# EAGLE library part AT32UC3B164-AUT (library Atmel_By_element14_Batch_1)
MCU
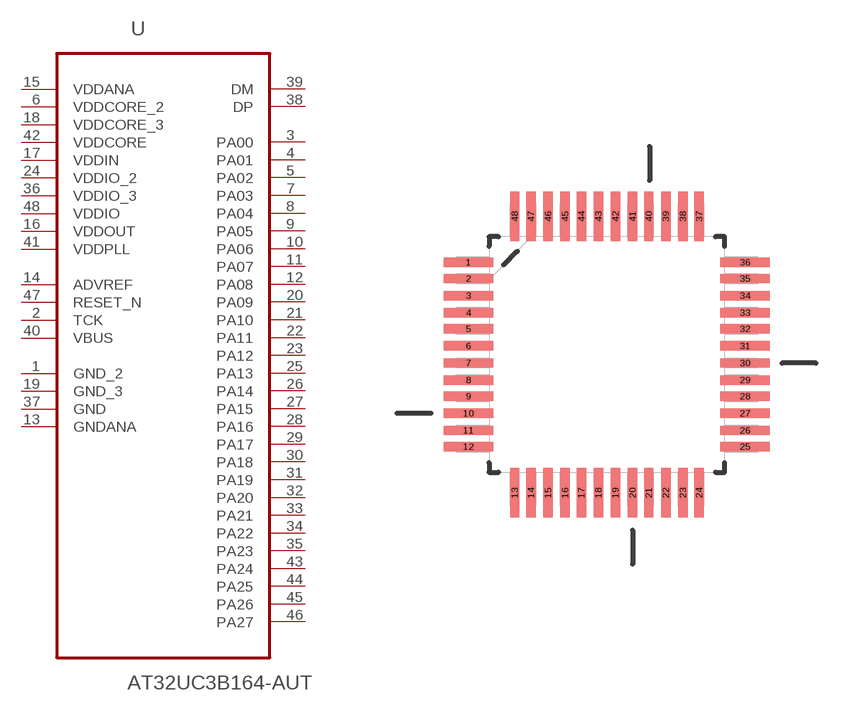
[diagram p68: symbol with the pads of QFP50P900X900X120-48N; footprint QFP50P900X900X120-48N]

Designator prefix U

## AT32UC3B164-AUT (DESCRIPTION: MCU; MPN: AT32UC3B164-AUT; OC_FARNELL: 1841642; OC_NEWARK: 12T1375; PACKAGE: QFP-48; SUPPLIER: Atmel)  [QFP50P900X900X120-48N]
1  GND_2  pas
2  TCK  in
3  PA00
4  PA01
5  PA02
6  VDDCORE_2  pwr
7  PA03
8  PA04
9  PA05
10  PA06
11  PA07
12  PA08
13  GNDANA  pas
14  ADVREF  in
15  VDDANA  pwr
16  VDDOUT  pwr
17  VDDIN  pwr
18  VDDCORE_3  pwr
19  GND_3  pas
20  PA09
21  PA10
22  PA11
23  PA12
24  VDDIO_2  pwr
25  PA13
26  PA14
27  PA15
28  PA16
29  PA17
30  PA18
31  PA19
32  PA20
33  PA21
34  PA22
35  PA23
36  VDDIO_3  pwr
37  GND  pas
38  DP
39  DM
40  VBUS  in
41  VDDPLL  pwr
42  VDDCORE  pwr
43  PA24
44  PA25
45  PA26
46  PA27
47  RESET_N  in
48  VDDIO  pwr

## Footprint QFP50P900X900X120-48N (pad centres in mm)
smd 1.473 x 0.279: 1 -4.115,2.743; 2 -4.115,2.261; 3 -4.115,1.753; 4 -4.115,1.245; 5 -4.115,0.762; 6 -4.115,0.254; 7 -4.115,-0.254; 8 -4.115,-0.762; 9 -4.115,-1.245; 10 -4.115,-1.753; 11 -4.115,-2.261; 12 -4.115,-2.743; 25 4.115,-2.743; 26 4.115,-2.261; 27 4.115,-1.753; 28 4.115,-1.245; 29 4.115,-0.762; 30 4.115,-0.254; 31 4.115,0.254; 32 4.115,0.762; 33 4.115,1.245; 34 4.115,1.753; 35 4.115,2.261; 36 4.115,2.743
smd 0.279 x 1.473: 13 -2.743,-4.115; 14 -2.261,-4.115; 15 -1.753,-4.115; 16 -1.245,-4.115; 17 -0.762,-4.115; 18 -0.254,-4.115; 19 0.254,-4.115; 20 0.762,-4.115; 21 1.245,-4.115; 22 1.753,-4.115; 23 2.261,-4.115; 24 2.743,-4.115; 37 2.743,4.115; 38 2.261,4.115; 39 1.753,4.115; 40 1.245,4.115; 41 0.762,4.115; 42 0.254,4.115; 43 -0.254,4.115; 44 -0.762,4.115; 45 -1.245,4.115; 46 -1.753,4.115; 47 -2.261,4.115; 48 -2.743,4.115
